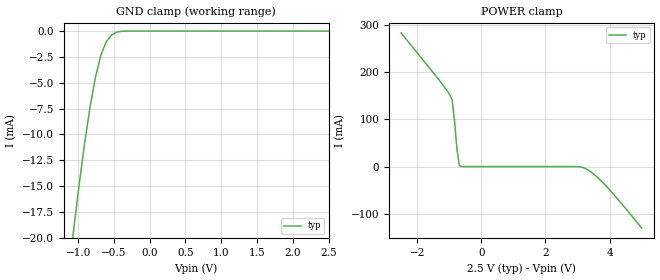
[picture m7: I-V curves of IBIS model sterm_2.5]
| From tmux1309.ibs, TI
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| sterm_2.5
[Model]   sterm_2.5
Model_type   Terminator
|   typ   min   max
C_comp   1.008417e-12   NA   NA
[Voltage Range]   2.5   NA   NA
[Temperature Range]   27   NA   NA
[Power Clamp Reference]   2.5   NA   NA
[GND Clamp Reference]   0   NA   NA
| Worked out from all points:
|   GND clamp passes 1 mA (typ) near -0.60 V on its own axis
|   POWER clamp passes 1 mA (typ) near -0.64 V on its own axis
[GND Clamp]
|   Voltage   I(typ)   I(min)   I(max)
-5V       -20.06kA   NA         NA
-1.061V   -19.14mA   NA         NA
-984.8mV  -14.81mA   NA         NA
-909.1mV  -10.85mA   NA         NA
-833.3mV  -7.351mA   NA         NA
-757.6mV  -4.455mA   NA         NA
-681.8mV  -2.33mA    NA         NA
-606.1mV  -1.022mA   NA         NA
-530.3mV  -349.6uA   NA         NA
-454.5mV  -84.89uA   NA         NA
-303mV    -1.843uA   NA         NA
2.5V      620.2pA    NA         NA
[POWER Clamp]
|   Voltage   I(typ)   I(min)   I(max)
-2.5V     282.7mA    NA         NA
-1.212V   174.1mA    NA         NA
-984.9mV  152.3mA    NA         NA
-909.1mV  141.4mA    NA         NA
-833.3mV  96.91mA    NA         NA
-757.6mV  36.54mA    NA         NA
-681.8mV  2.121mA    NA         NA
-606.1mV  25.25uA    NA         NA
3.182V    -2.33mA    NA         NA
3.485V    -14.81mA   NA         NA
3.864V    -39.13mA   NA         NA
5V        -130.1mA   NA         NA
